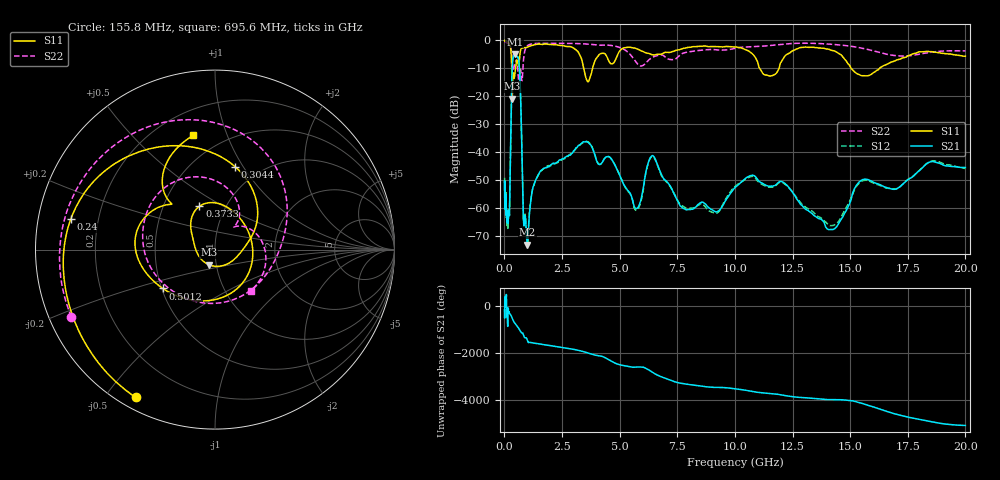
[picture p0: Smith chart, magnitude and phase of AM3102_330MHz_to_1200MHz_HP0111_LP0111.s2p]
! Date/Time: Tue, Sep 11, 2018 5:16 PM
! Network Analyzer: Agilent Technologies E8362B Rev: A.07.50.63
! Sweep from 0.010 to 20.000 GHz, 1601 Points, Sweep Type: LOG
! Power Supply: 4.949 V, 0.001 A
# Hz S DB R 50
!freq MagS11 AngS11 MagS21 AngS21 MagS12 AngS12 MagS22 AngS22
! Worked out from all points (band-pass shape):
!   1601 points, 10 MHz to 20 GHz, reference 50 ohm
!   highest |S21| = -4.87 dB at 449.3 MHz (marker M1); lowest = -73.2 dB at 993.4 MHz (marker M2)
!   |S21| within 3 dB of the highest: 353.6 MHz to 633.7 MHz (280.1 MHz wide, 56.7 % of centre)
!   lowest |S11| = -20.8 dB at 341.1 MHz (marker M3), VSWR 1.20, Z = 46 - j7.81 ohm
!   |S11| at or under -10 dB: 3.44 GHz to 3.824 GHz (383.9 MHz wide, 10.6 % of centre); 11.08 GHz to 11.92 GHz (841.1 MHz wide, 7.32 % of centre); 15.04 GHz to 16.28 GHz (1.232 GHz wide, 7.87 % of centre)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
!   |S22| runs from -15.7 to -0.2 dB; largest |S21 - S12| = 0.0093
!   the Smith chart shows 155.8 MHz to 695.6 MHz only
!   S11 on the Smith chart (normalised r, x): 155.8 MHz: 0.05, -0.60; 240 MHz: 0.10, +0.10; 304.4 MHz: 0.77, +0.92; 373.3 MHz: 0.75, +0.39; 501.2 MHz: 0.51, -0.25; 695.6 MHz: 0.35, +0.77
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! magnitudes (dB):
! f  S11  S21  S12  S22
! 10 MHz  0.0  -50.4  -49.2  -0.2
! 35.55 MHz  0.0  -59.0  -59.2  -0.4
! 126.4 MHz  -0.4  -63.1  -65.9  -0.9
! 155.8 MHz  -0.6  -64.0  -65.6  -1.1
! 240 MHz  -1.7  -52.4  -52.8  -1.7
! 304.4 MHz  -6.5  -21.1  -21.2  -3.8
! 341.1 MHz  -20.8  -9.6  -9.7  -8.1
! 373.3 MHz  -11.8  -6.4  -6.5  -10.5
! 447.2 MHz  -12.6  -4.9  -4.9  -8.5
! 449.3 MHz  -12.4  -4.9  -4.9  -8.5
! 501.2 MHz  -8.8  -5.1  -5.3  -7.2
! 695.6 MHz  -3.8  -18.2  -18.2  -10.3
! 829.3 MHz  -2.6  -64.5  -64.5  -7.0
! 993.4 MHz  -2.4  -73.2  -73.5  -1.9
! 1.59 GHz  -1.4  -46.6  -46.6  -1.0
! 3.582 GHz  -14.3  -36.3  -36.2  -1.3
! 5.652 GHz  -2.7  -59.7  -60.4  -7.1
! 6.457 GHz  -5.2  -41.4  -41.6  -5.9
! 7.845 GHz  -2.7  -60.4  -59.9  -4.3
! 10.73 GHz  -4.6  -48.3  -48.7  -2.3
! 14.14 GHz  -3.4  -67.7  -66.3  -1.3
! 20 GHz  -5.7  -45.5  -45.8  -3.7
